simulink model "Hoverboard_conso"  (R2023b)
settings: Solver=ode15s  StartTime=0.0  FixedStep=0.001  RelTol=1e-3
libraries: fl_lib x13, nesl_utility x7, batteryecm_lib x1, ee_lib x1

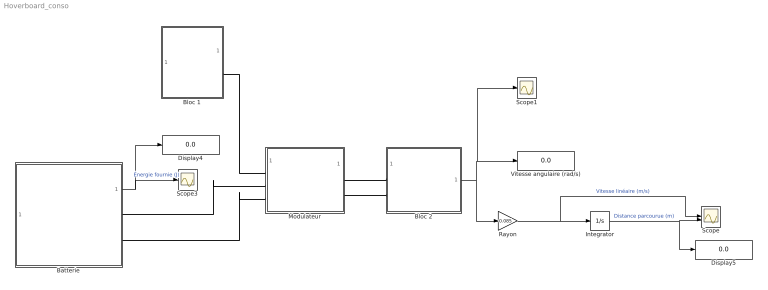
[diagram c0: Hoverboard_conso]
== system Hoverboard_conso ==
  Batterie : Subsystem  mask{Vn=12, Cbc=50000, Vd=11.5, Cbd=25000, Rb=0.02}
      mask prompts: Vn "Tension chargée (V)"; Cbc "Capacité (mAh)"; Vd "Tension déchargée (V)"; Cbd "Capacité déchargée (mAh)"; Rb "Résistance interne (Ohm)"
  Bloc 1 : Subsystem  mask{alpha=0}
      mask prompts: alpha "Angle d'inclinaison (°)"
  Bloc 2 : Subsystem  mask{R=5, Kc=0.4, Co=0.06, fm=0.0085, Mh=10, Mu=0}
      mask prompts: R "Résistance (Ohm)"; Kc "Constante de couple (Nm/A)"; Co "Couple sec (Nm)"; fm "Frottement visqueux (Nm.s/rad)"; Mh "Masse de l'hoverboard (Kg)"; Mu "Masse de l'utilisateur (Kg)"
  Display4 : Display
  Display5 : Display
  Integrator : Integrator
  Modulateur : Subsystem
  Rayon : Gain  Gain=0.085
  Scope : Scope  NumInputPorts=2
  Scope1 : Scope
  Scope3 : Scope
  Vitesse angulaire (rad/s) : Display
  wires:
  Integrator/1 -> Display5/1, Scope/2  "Distance parcourue (m)"
  Rayon/1 -> Integrator/1, Scope/1  "Vitesse linéaire (m/s)"
  Batterie/1(Batterie2) -> Display4/1, Scope3/1  "Énergie fournie (J)"
  Bloc 2/1(Omega) -> Rayon/1, Scope1/1, Vitesse angulaire (rad/s)/1
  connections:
  Batterie/RConn1 -- Modulateur/LConn2
  Batterie/RConn2 -- Modulateur/LConn3
  Modulateur/RConn2 -- Bloc 2/LConn2
  Modulateur/RConn1 -- Bloc 2/LConn1
  Bloc 1/RConn1 -- Modulateur/LConn1

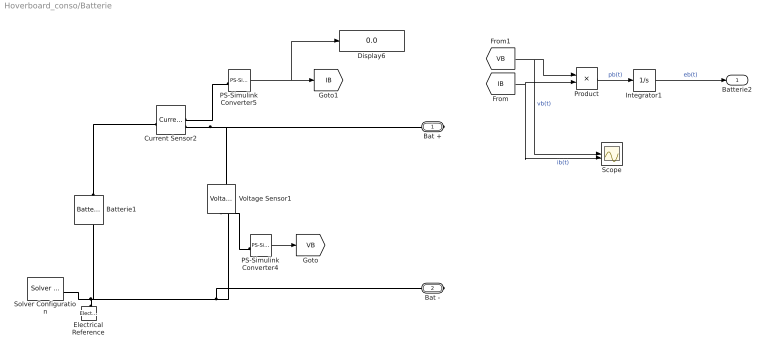
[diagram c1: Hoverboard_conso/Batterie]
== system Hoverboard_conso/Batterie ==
  Batterie1 : batteryecm_lib/Battery  Vnom=Vn V  prm_dir=simscape.enum.battery.prm_dir.disabled  R1_dis=2 Ohm  R1_ch=2 Ohm  R1=Rb Ohm  prm_AH=2  AH=Cbc mAh  V1=Vd V  AH1=Cbd mAh  prm_R2=1  R2=2000 Ohm  Tmeas=298.15 K  charge_measurement_port=simscape.enum.battery.enable.no  prm_dyn=1  Rp1=0.005 Ohm  tau1=30 s  Rp2=0.005 Ohm  tau2=30 s  Rp3=0.005 Ohm  tau3=30 s  Rp4=0.005 Ohm  tau4=30 s  Rp5=0.005 Ohm  tau5=30 s  prm_fade=1  N_fade=100  AH_fade=45 hr*A  R1_fade=2.02 Ohm  R1_ch_fade=2.02 Ohm  V1_fade=10.35 V  prm_age=simscape.enum.battery.prm_age.disabled  prm_age_OCV=simscape.enum.battery.prm_age_OCV.OCV  OCV_age=0.9  SOC_age=60  Tmeas_age=298.15 K  delta_time_age_vec=[0] d  temperature_age_vec=[273] K  OCV_scaling_age=2.2134e6  OCV_offset_age=1.632e6  temp_exp_age=0.515833569 V  t_exp_age=0.75  Vnom_T2=12 V  R1_T2=2.2 Ohm  R1_T2_dis=2.2 Ohm  R1_T2_ch=2.2 Ohm  V1_T2=11.4 V  R2_T2=2200 Ohm  Rp1_T2=0.005 Ohm  tau1_T2=30 s  Rp2_T2=0.005 Ohm  tau2_T2=30 s  Rp3_T2=0.005 Ohm  tau3_T2=30 s  Rp4_T2=0.005 Ohm  tau4_T2=30 s  Rp5_T2=0.005 Ohm  tau5_T2=30 s  Tmeas2=273.15 K  thermal_port=simscape.enum.thermaleffects.omit  thermal_mass=30000 J/K  i_specify=off  i_priority=None  i=0 A  i_nominal_specify=off  i_nominal_unit=A  i_nominal_value=1  v_specify=off  v_priority=None  v=0 V  v_nominal_specify=off  v_nominal_unit=V  v_nominal_value=1  charge_specify=off  charge_priority=High  charge=50 hr*A  charge_nominal_specify=off  charge_nominal_unit=A*hr  charge_nominal_value=1  num_cycles_specify=off  num_cycles_priority=High  num_cycles=0  num_cycles_nominal_specify=off  num_cycles_nominal_unit=1  num_cycles_nominal_value=1  temperature_specify=off  temperature_priority=High  temperature=298.15 K  temperature_nominal_specify=off  temperature_nominal_unit=K  temperature_nominal_value=1
  Current Sensor2 : fl_lib/Electrical/Electrical Sensors/Current Sensor
  Display6 : Display
  Electrical Reference : fl_lib/Electrical/Electrical Elements/Electrical Reference
  Integrator1 : Integrator
  PS-Simulink Converter4 : nesl_utility/PS-Simulink Converter  PhysicalDomain=network_engine_domain  SubClassName=ps_output  LeftPortType=input  RightPortType=output  PseudoPeriodic=off  Frequencies=[]  VectorFormat=1-D array  Unit=V  AffineConversion=off
  PS-Simulink Converter5 : nesl_utility/PS-Simulink Converter  PhysicalDomain=network_engine_domain  SubClassName=ps_output  LeftPortType=input  RightPortType=output  PseudoPeriodic=off  Frequencies=[]  VectorFormat=1-D array  Unit=A  AffineConversion=off
  Product : Product
  Scope : Scope  NumInputPorts=2
  Solver Configuration : nesl_utility/Solver Configuration  PhysicalDomain=network_engine_domain  SubClassName=solver  LeftPortType=input  RightPortType=generic  Tones=[]  Harmonics=[]  SimulateNoise=off  Profile=off  UseLocalSampling=off  EnableSwitchedLinearOptims=on  FrequencyDomain=off  UseCCode=off  RelTol=0.001  AbsTol=1e-06  MinStep=1e-09  ToWorkspace=off  RevertToSquareIcSolve=off  NumHomotopyIterations=100  PhasorMode=off  PhasorModeNumHarmonics=1  ConsistencySolver=NEWTON_FTOL  IndexReductionMethod=DerivativeReplacement  DoDC=off  ResidualTolerance=1e-09  ConsistencyTolSource=GLOBAL  ConsistencyAbsTol=0.001  ConsistencyRelTol=0.001  ConsistencyTolFactor=0.001  UseLocalSolver=off  LocalSolverChoice=NE_BACKWARD_EULER_ADVANCER  ResolveIndetEquations=on  FunctionEvalNumThread=1  LocalSolverSampleTime=0.001  DoFixedCost=off  MaxNonlinIter=3  MaxModeIter=2  ComputeImpulses=off  ImpulseIterations=2  LinearAlgebra=Sparse  LinearAlgebraNumThread=0  EquationFormulation=NE_TIME_EF  DelaysMemoryBudget=1024  AutomaticFiltering=on  FilteringTimeConstant=0.001  PartitionStorageMethod=AS_NEEDED  PartitionMemoryBudget=1024  PartitionMethod=FAST  MultibodyUseLocalSolver=off  MultibodyLocalSolverChoice=ODE1  MultibodyLocalSolverSampleTime=0.001
  Voltage Sensor1 : fl_lib/Electrical/Electrical Sensors/Voltage Sensor
  Bat + : PMIOPort  Side=Right
  Bat - : PMIOPort  Port=2  Side=Right
  Batterie2 : Outport  VectorParamsAs1DForOutWhenUnconnected=off
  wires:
  [VB] -> Scope/1, Product/1  "vb(t)"
  PS-Simulink Converter5/1 -> [IB], Display6/1
  [IB] -> Scope/2, Product/2  "ib(t)"
  PS-Simulink Converter4/1 -> [VB]
  Integrator1/1 -> Batterie2/1  "eb(t)"
  Product/1 -> Integrator1/1  "pb(t)"
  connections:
  Electrical Reference/LConn1 -- Batterie1/RConn1 -- Solver Configuration/RConn1 -- Bat -/RConn1 -- Voltage Sensor1/RConn2
  Current Sensor2/RConn2 -- Bat +/RConn1 -- Voltage Sensor1/LConn1
  Batterie1/LConn1 -- Current Sensor2/LConn1
  PS-Simulink Converter5/LConn1 -- Current Sensor2/RConn1
  PS-Simulink Converter4/LConn1 -- Voltage Sensor1/RConn1

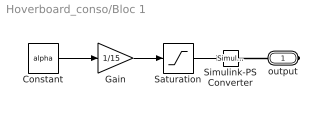
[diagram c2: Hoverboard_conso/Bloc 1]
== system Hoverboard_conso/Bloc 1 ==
  Constant : Constant  Value=alpha
  Gain : Gain  Gain=1/15
  Saturation : Saturate  UpperLimit=0.95  LowerLimit=0
  Simulink-PS Converter : nesl_utility/Simulink-PS Converter  PhysicalDomain=network_engine_domain  SubClassName=ps_input  LeftPortType=input  RightPortType=output  PseudoPeriodic=off  Frequencies=[]  NoiseDistribution=none  NoiseParameters=[]  Unit=1  AffineConversion=off  FilteringAndDerivatives=provide  SimscapeFilterOrder=1  InputFilterTimeConstant=0.001  UdotUserProvided=0
  output : PMIOPort  Side=Right
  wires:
  Saturation/1 -> Simulink-PS Converter/1
  Gain/1 -> Saturation/1
  Constant/1 -> Gain/1
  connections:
  Simulink-PS Converter/RConn1 -- output/RConn1

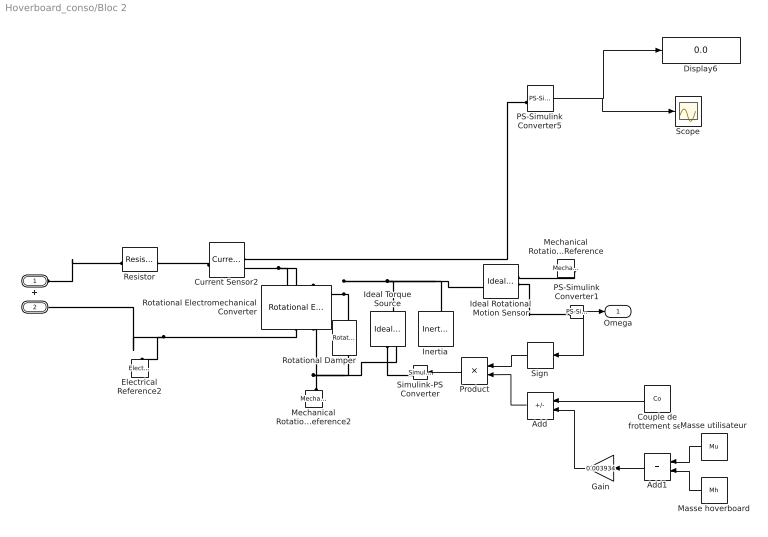
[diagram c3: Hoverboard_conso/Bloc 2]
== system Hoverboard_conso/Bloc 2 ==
  Add : Sum  Inputs=--
  Add1 : Sum
  Couple de frottement sec : Constant  Value=Co
  Current Sensor2 : fl_lib/Electrical/Electrical Sensors/Current Sensor
  Display6 : Display
  Electrical Reference2 : fl_lib/Electrical/Electrical Elements/Electrical Reference
  Gain : Gain  Gain=0.003934
  Ideal Rotational Motion Sensor : fl_lib/Mechanical/Mechanical Sensors/Ideal Rotational Motion Sensor  reference=foundation.enum.MeasurementReference.difference  acceleration_port=false  velocity_port=true  position_port=true  wrap_angle=false  offset=0 rad
  Ideal Torque Source : fl_lib/Mechanical/Mechanical Sources/Ideal Torque Source
  Inertia : fl_lib/Mechanical/Rotational Elements/Inertia  inertia=0.01 g*cm^2  num_ports=foundation.enum.numPorts2.one  w_specify=off  w_priority=High  w=0 rad/s  w_nominal_specify=off  w_nominal_unit=rad/s  w_nominal_value=1  t_specify=off  t_priority=High  t=0 N*m  t_nominal_specify=off  t_nominal_unit=N*m  t_nominal_value=1
  Masse hoverboard : Constant  Value=Mh
  Masse utilisateur : Constant  Value=Mu
  Mechanical Rotational Reference : fl_lib/Mechanical/Rotational Elements/Mechanical Rotational Reference
  Mechanical Rotational Reference2 : fl_lib/Mechanical/Rotational Elements/Mechanical Rotational Reference
  PS-Simulink Converter1 : nesl_utility/PS-Simulink Converter  PhysicalDomain=network_engine_domain  SubClassName=ps_output  LeftPortType=input  RightPortType=output  PseudoPeriodic=off  Frequencies=[]  VectorFormat=1-D array  Unit=rad/s  AffineConversion=off
  PS-Simulink Converter5 : nesl_utility/PS-Simulink Converter  PhysicalDomain=network_engine_domain  SubClassName=ps_output  LeftPortType=input  RightPortType=output  PseudoPeriodic=off  Frequencies=[]  VectorFormat=1-D array  Unit=A  AffineConversion=off
  Product : Product
  Resistor : fl_lib/Electrical/Electrical Elements/Resistor  R=R Ohm  i_specify=off  i_priority=None  i=0 A  i_nominal_specify=off  i_nominal_unit=A  i_nominal_value=1  v_specify=off  v_priority=None  v=0 V  v_nominal_specify=off  v_nominal_unit=V  v_nominal_value=1
  Rotational Electromechanical Converter : fl_lib/Electrical/Electrical Elements/Rotational Electromechanical Converter  K=Kc V/(rad/s)  i_specify=off  i_priority=None  i=0 A  i_nominal_specify=off  i_nominal_unit=A  i_nominal_value=1  v_specify=off  v_priority=None  v=0 V  v_nominal_specify=off  v_nominal_unit=V  v_nominal_value=1  t_specify=off  t_priority=None  t=0 N*m  t_nominal_specify=off  t_nominal_unit=N*m  t_nominal_value=1  w_specify=off  w_priority=None  w=0 rad/s  w_nominal_specify=off  w_nominal_unit=rad/s  w_nominal_value=1
  Rotational Damper : fl_lib/Mechanical/Rotational Elements/Rotational Damper  D=fm N*m/(rad/s)  w_specify=off  w_priority=None  w=0 rad/s  w_nominal_specify=off  w_nominal_unit=rad/s  w_nominal_value=1  t_specify=off  t_priority=None  t=0 N*m  t_nominal_specify=off  t_nominal_unit=N*m  t_nominal_value=1
  Scope : Scope
  Sign : Signum
  Simulink-PS Converter : nesl_utility/Simulink-PS Converter  PhysicalDomain=network_engine_domain  SubClassName=ps_input  LeftPortType=input  RightPortType=output  PseudoPeriodic=off  Frequencies=[]  NoiseDistribution=none  NoiseParameters=[]  Unit=1  AffineConversion=off  FilteringAndDerivatives=provide  SimscapeFilterOrder=1  InputFilterTimeConstant=0.001  UdotUserProvided=0
  + : PMIOPort  Side=Left
  - : PMIOPort  Port=2  Side=Left
  Omega : Outport  VectorParamsAs1DForOutWhenUnconnected=off
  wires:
  PS-Simulink Converter1/1 -> Sign/1, Omega/1
  Add1/1 -> Gain/1
  Masse utilisateur/1 -> Add1/1
  Masse hoverboard/1 -> Add1/2
  Gain/1 -> Add/2
  Couple de frottement sec/1 -> Add/1
  PS-Simulink Converter5/1 -> Scope/1, Display6/1
  Product/1 -> Simulink-PS Converter/1
  Add/1 -> Product/2
  Sign/1 -> Product/1
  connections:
  +/RConn1 -- Resistor/LConn1
  Rotational Electromechanical Converter/LConn2 -- Inertia/LConn1 -- Ideal Rotational Motion Sensor/LConn1 -- Ideal Torque Source/LConn1 -- Rotational Damper/LConn1
  Mechanical Rotational Reference2/LConn1 -- Rotational Damper/RConn1 -- Ideal Torque Source/RConn2 -- Rotational Electromechanical Converter/RConn2
  Rotational Electromechanical Converter/RConn1 -- Electrical Reference2/LConn1 -- -/RConn1
  Ideal Torque Source/RConn1 -- Simulink-PS Converter/RConn1
  Ideal Rotational Motion Sensor/RConn2 -- PS-Simulink Converter1/LConn1
  Mechanical Rotational Reference/LConn1 -- Ideal Rotational Motion Sensor/RConn1
  Current Sensor2/RConn2 -- Rotational Electromechanical Converter/LConn1
  PS-Simulink Converter5/LConn1 -- Current Sensor2/RConn1
  Current Sensor2/LConn1 -- Resistor/RConn1

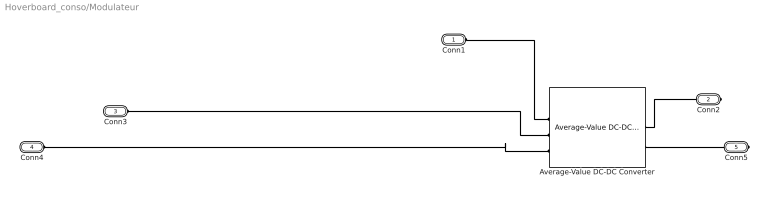
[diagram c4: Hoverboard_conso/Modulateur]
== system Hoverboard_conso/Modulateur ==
  Average-Value DC-DC Converter : ee_lib/Semiconductors & Converters/Converters/Average-Value DC-DC Converter  control_option=ee.enum.converters.controlinput.dutycycle  converter_type=ee.enum.converters.dcdctype.buckboost  efficiency_option=ee.enum.converters.efficiency.constant  efficiency_fixed=90  i_vec=[0, 2, 5] A  efficiency_vec=[90, 95, 98]
  Conn1 : PMIOPort  Side=Left
  Conn2 : PMIOPort  Port=2  Side=Right
  Conn3 : PMIOPort  Port=3  Side=Left
  Conn4 : PMIOPort  Port=4  Side=Left
  Conn5 : PMIOPort  Port=5  Side=Right
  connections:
  Average-Value DC-DC Converter/RConn1 -- Conn2/RConn1
  Average-Value DC-DC Converter/LConn2 -- Conn3/RConn1
  Average-Value DC-DC Converter/LConn1 -- Conn1/RConn1
  Average-Value DC-DC Converter/LConn3 -- Conn4/RConn1
  Average-Value DC-DC Converter/RConn2 -- Conn5/RConn1
